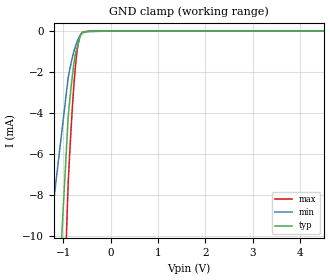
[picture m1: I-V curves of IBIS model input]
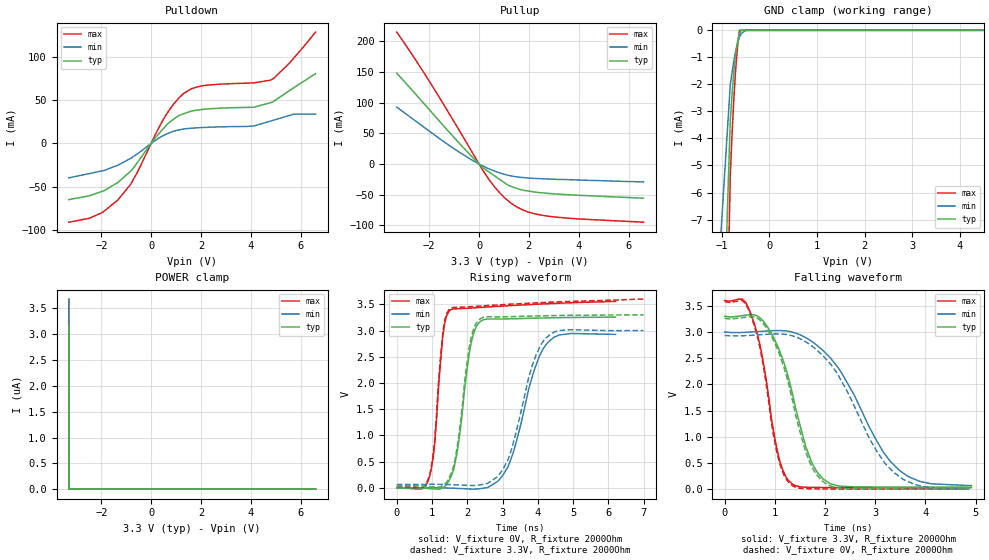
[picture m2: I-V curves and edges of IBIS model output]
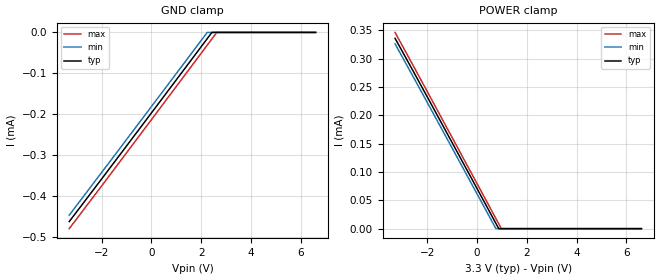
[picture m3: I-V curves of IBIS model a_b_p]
|Texas Instruments Incorporated
| Low-Voltage High-Speed Quadruple Differential Line Receiver
| With +/-15-kV IEC ESD
| Marketing part#   Digital Voltage Range   Package-type   #pins
| AM26LV32EIPWR   3.0V-3.6V   TSSOP   16
| AM26LV32EIPWRG4   3.0V-3.6V   TSSOP   16
| AM26LV32EIRGYR   3.0V-3.6V   VQFN   16
| AM26LV32EIRGYRG4   3.0V-3.6V   VQFN   16
| AM26LV32EID   3.0V-3.6V   SOIC   16
| AM26LV32EIDR   3.0V-3.6V   SOIC   16
[IBIS Ver]   4.1
[File name]   am26lv32e.ibs
[File Rev]   1.1
[Date]   11/01/2018
[Source]
| Texas Instruments Incorporated.
| Central Analog Engineering
| 12500 TI Blvd
| Dallas, TX -75243
[Notes]   Revision History:
| Rev 1.1: 11/01/2018
| - Add D package component
| Rev 1.0: 6/13/2013
| - Initial version of the model
| - Model generated from simulations in TISPICE
| - Model matched to SPICE simulation
| - C_comp although listed in numerical order of value are
|   obtained from varying PVT conditions. For PVT conditions for
|   each specific value refer the buffer description under
|   respective [Model]. IBIS model user is responsible for using
|   appropriate C_comp to simulate for Signal Integrity.
|*  EXCEPTION:   *
|*  - For model a_b_p and a_b_n ,There will be leakage in POWER Clamp   *
|*   IV table because of resistors R5,R14 connected to pad and GND Clamp   *
|*   IV table because of resistor R9 Connected to PAD.   *
|*  MODEL NOTE   *
|*  - This model is provided for use with both AM26LV32E and AM26LV32   *
|*   The silicon processes are different between these two parts, but only *
|*   one model is provided. The model is based on the AM26LV32E   *
|*   The accuracy of this model for AM26LV32 is limited and cannot be   *
|*   assured.
[Disclaimer]
| This model is designed as an aid for customers of Texas Instruments.
| TI and its licensors and suppliers make no warranties, either expressed
| or implied, with respect to this  model, including the warranties of
| merchantability or fitness for a particular purpose. The model is
| provided solely on an "as is" basis. The entire risk as to its quality
| and performance is with the customer.
[Copyright]
(C) Copyright 2018 Texas Instruments Incorporated.All rights reserved.
|   AM26LV32EPW
[Component]   AM26LV32EPW
[Manufacturer]   TI
[Package]   |16 TSSOP  -  PW  package
|   typ   min   max
R_pkg   0.19278   0.17677   0.20396
L_pkg   2.52752nH   2.29134nH   3.00408nH
C_pkg   0.42124pF   0.37067pF   0.48718pF
[Pin]  signal_name   model_name   R_pin   L_pin   C_pin
1   1B   a_b_n   0.17681   3.00040nH  0.48133pF
2   1A   a_b_p   0.19015   2.64657nH  0.48718pF
3   1Y   output   0.20396   2.39994nH  0.37179pF
4   G   input   0.19498   2.32104nH  0.37697pF
5   2Y   output   0.19142   2.29222nH  0.37501pF
6   2A   a_b_p   0.20200   2.38573nH  0.37069pF
7   2B   a_b_n   0.19014   2.64482nH  0.48580pF
8   GND   gnd   0.17006   2.94878nH  0.47879pF
9   3B   a_b_n   0.17677   3.00408nH  0.48145pF
10   3A   a_b_p   0.19010   2.64442nH  0.48578pF
11   3Y   output   0.20396   2.40233nH  0.37179pF
12   _G   input   0.19498   2.32182nH  0.37695pF
13   4Y   output   0.19142   2.29134nH  0.37502pF
14   4A   a_b_p   0.20200   2.38374nH  0.37067pF
15   4B   a_b_n   0.19019   2.64687nH  0.48695pF
16   VCC   power   0.18007   3.02750nH  0.48186pF
[Diff_pin]   inv_pin   vdiff   tdelay_typ   tdelay_min   tdelay_max
2   1   0.4   NA   NA   NA
6   7   0.4   NA   NA   NA
10   9   0.4   NA   NA   NA
14   15   0.4   NA   NA   NA
|   AM26LV32ERGY
[Component]   AM26LV32ERGY
[Manufacturer]   TI
[Package]   |16 VQFN   -  RGY package
|   typ   min   max
R_pkg   0.07133   0.06853   0.07388
L_pkg   1.07820nH   1.02485nH   1.12558nH
C_pkg   0.21525pF   0.20251pF   0.22285pF
[Pin]  signal_name   model_name   R_pin   L_pin   C_pin
1   1B   a_b_n   0.07388   1.12180nH  0.20251pF
2   1A   a_b_p   0.07293   1.10260nH  0.21277pF
3   1Y   output   0.07064   1.06987nH  0.22157pF
4   G   input   0.06991   1.04900nH  0.21124pF
5   2Y   output   0.06853   1.03338nH  0.20945pF
6   2A   a_b_p   0.07048   1.05873nH  0.22115pF
7   2B   a_b_n   0.07292   1.10180nH  0.22284pF
8   GND   gnd   0.07165   1.08613nH  0.22006pF
9   3B   a_b_n   0.07388   1.12558nH  0.21274pF
10   3A   a_b_p   0.07293   1.11070nH  0.21297pF
11   3Y   output   0.07064   1.06167nH  0.22136pF
12   _G   input   0.06991   1.05770nH  0.21146pF
13   4Y   output   0.06853   1.02485nH  0.20922pF
14   4A   a_b_p   0.07048   1.06724nH  0.22135pF
15   4B   a_b_n   0.07292   1.10994nH  0.22285pF
16   VCC   power   0.07593   1.15699nH  0.21430pF
[Diff_pin]   inv_pin   vdiff   tdelay_typ   tdelay_min   tdelay_max
2   1   0.4   NA   NA   NA
6   7   0.4   NA   NA   NA
10   9   0.4   NA   NA   NA
14   15   0.4   NA   NA   NA
|   AM26LV32EID
[Component]   AM26LV32EID
[Manufacturer]   TI
[Package]   |16 SOIC  -  D  package
|   typ   min   max
R_pkg   0.1097   0.0876   0.1214
L_pkg   2.6739n   1.8660n   3.6087n
C_pkg   0.5144p   0.3762p   0.7307p
[Pin]  signal_name   model_name   R_pin   L_pin   C_pin
1   1B   a_b_n   0.12139  3.60868n  0.72658p
2   1A   a_b_p   0.11814  2.95593n  0.55477p
3   1Y   output   0.11472  2.32743n  0.39842p
4   G   input   0.08877  1.89317n  0.37966p
5   2Y   output   0.08774  1.87902n  0.37623p
6   2A   a_b_p   0.11080  2.26165n  0.39561p
7   2B   a_b_n   0.11803  2.94830n  0.55794p
8   GND   gnd   0.11660  3.51494n  0.72633p
9   3B   a_b_n   0.12090  3.58634n  0.73071p
10   3A   a_b_p   0.11796  2.94490n  0.55767p
11   3Y   output   0.11472  2.32235n  0.39894p
12   _G   input   0.08886  1.88922n  0.37773p
13   4Y   output   0.08764  1.86597n  0.37772p
14   4A   a_b_p   0.11080  2.25473n  0.39472p
15   4B   a_b_n   0.11821  2.95453n  0.55408p
16   VCC   power   0.11952  3.57518n  0.72334p
[Diff_pin]   inv_pin   vdiff   tdelay_typ   tdelay_min   tdelay_max
2   1   0.4   NA   NA   NA
6   7   0.4   NA   NA   NA
10   9   0.4   NA   NA   NA
14   15   0.4   NA   NA   NA
| Models and submodels in the file (4): input (Input), output (3-state), a_b_p (Input), a_b_n (Input)
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|   input Model
[Model]   input
Model_type   Input
Vinl = 0.8
Vinh = 2.0
|   typ   min   max
|   (nom PVT)   (fast PVT)   (slow PVT)
C_comp   2.118e-12   2.106e-12   2.143e-12
| Where nom  PVT is Nominal Process, 3.3V, 27C
|   Fast PVT is Strong Process,  3.6V, -40C
|   Slow PVT is Weak Process,   3V, 125C
[Voltage Range]   3.3   3   3.6
|Junction Temperature
[Temperature Range]   27   125   -40
[Power Clamp Reference]   3.3   3   3.6
[GND Clamp Reference]   0   0   0
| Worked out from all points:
|   GND clamp passes 1 mA (typ) near -0.73 V on its own axis
[GND Clamp]
|   Voltage   I(typ)   I(min)   I(max)
-3.3V     -815.5mA   -63.93mA   -1.464A
-1.77V    -41.57mA   -19.44mA   -66.75mA
-897.6mV  -4.201mA   -2.276mA   -7.453mA
-853.2mV  -3.129mA   -1.753mA   -5.46mA
-810mV    -2.207mA   -1.299mA   -3.763mA
-774mV    -1.556mA   -971.7uA   -2.552mA
-738mV    -1.048mA   -694.3uA   -1.568mA
-702mV    -744.7uA   -469.8uA   -844.2uA
-669.6mV  -471.9uA   -316uA     -422.3uA
-633.6mV  -168.7uA   -195.4uA   -167.8uA
-586.8mV  -59.62uA   -89.39uA   -42.05uA
6.6V      0A         0A         0A
[POWER Clamp]
|   Voltage   I(typ)   I(min)   I(max)
-3.3V     0A         0A         0A
0V        0A         0A         0A
6.6V      0A         0A         0A
|   output Model
[Model]   output
Model_type   3-state
Polarity   Inverting
Vmeas = 1.65
Vref = 0
Cref = 15pF
Rref = 2000
|   typ   min   max
|   (nom PVT)   (fast PVT)   (slow PVT)
C_comp   3.751e-12   3.557e-12   4.057e-12
| Where nom  PVT is Nominal Process, 3.3V, 27C
|   Fast PVT is Strong Process,  3.6V, -40C
|   Slow PVT is Weak Process,   3V, 125C
[Voltage Range]   3.3   3   3.6
|Junction Temperature
[Temperature Range]   27   125   -40
[Pullup Reference]   3.3   3   3.6
[Pulldown Reference]   0   0   0
[Power Clamp Reference]   3.3   3   3.6
[GND Clamp Reference]   0   0   0
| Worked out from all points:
|   slope of the pulldown table from 0 to 0.495 V, typ, clamps not added: 28.7 ohm
|   slope of the pullup table from 0 to 0.495 V, typ, clamps not added: 31.5 ohm
|   GND clamp passes 1 mA (typ) near -0.72 V on its own axis
|   falling waveform, V_fixture 3.3V, R_fixture 2000Ohm: 20-80 % time 574ps typ, 1.02ns min, 377ps max; typ from 3.3 V to 0.038 V
|   rising waveform, V_fixture 0V, R_fixture 2000Ohm: 20-80 % time 363ps typ, 696ps min, 242ps max; typ from 0 V to 3.26 V
|   rising waveform, V_fixture 3.3V, R_fixture 2000Ohm: 20-80 % time 358ps typ, 671ps min, 246ps max; typ from 0.037 V to 3.3 V
|   falling waveform, V_fixture 0V, R_fixture 2000Ohm: 20-80 % time 563ps typ, 985ps min, 373ps max; typ from 3.26 V to 0 V
[Pulldown]
|   Voltage   I(typ)   I(min)   I(max)
-3.3V     -64.91mA   -39.78mA   -90.98mA
-2.486V   -60.54mA   -34.86mA   -86.52mA
-1.961V   -55.37mA   -31.68mA   -79.88mA
-1.345V   -45.31mA   -25.32mA   -65.66mA
-823.2mV  -32.07mA   -17.37mA   -47.39mA
584.4mV   20.16mA    10.34mA    32.12mA
1.312V    34.3mA     16.66mA    57.78mA
2.071V    39.2mA     18.38mA    66.61mA
4.125V    41.86mA    20.19mA    69.94mA
4.786V    47.01mA    25.76mA    73.04mA
5.742V    64.62mA    33.9mA     99.12mA
6.6V      80.6mA     33.9mA     128.6mA
[GND Clamp]
|   Voltage   I(typ)   I(min)   I(max)
-3.3V     -851.8mA   -106.7mA   -1.503A
-2.238V   -82.98mA   -41.6mA    -127.3mA
-825mV    -3.375mA   -2.041mA   -5.51mA
-801.6mV  -2.77mA    -1.749mA   -4.443mA
-776.4mV  -2.142mA   -1.436mA   -3.479mA
-749.1mV  -1.508mA   -1.138mA   -2.56mA
-726mV    -1.119mA   -890.4uA   -1.874mA
-675.6mV  -477.1uA   -503.2uA   -698.4uA
-628.8mV  -129.1uA   -249.4uA   0A
-597.3mV  -518.8nA   -135.5uA   0A
-498mV    -432.6nA   -2.253uA   0A
6.6V      0A         0A         0A
[Pullup]
|   Voltage   I(typ)   I(min)   I(max)
-3.3V     148mA      92.72mA    215mA
-2.17V    96.59mA    58.75mA    146.2mA
-825mV    35.29mA    20.19mA    57mA
19.8mV    -787.1uA   -413uA     -1.283mA
400.8mV   -13.03mA   -7.878mA   -25.36mA
850.8mV   -25.77mA   -14.78mA   -47.91mA
1.29V     -36.59mA   -19.41mA   -63.98mA
1.52V     -39.95mA   -20.98mA   -70.12mA
1.995V    -44.22mA   -22.92mA   -78.54mA
2.622V    -47.36mA   -24.22mA   -84.21mA
4.123V    -51.27mA   -26.26mA   -89.85mA
6.6V      -55.74mA   -29.32mA   -94.86mA
[POWER Clamp]
|   Voltage   I(typ)   I(min)   I(max)
-3.3V     3.161uA    3.682uA    3.68uA
-3.297V   1.724uA    545.5nA    2.147uA
-3.293V   0A         218.2nA    306.6nA
-3.293V   0A         163.7nA    0A
-3.291V   0A         0A         0A
6.6V      0A         0A         0A
[Ramp]
R_load = 2000
|   typ   min   max
dV/dt_r   1.95542/3.608e-10   1.75784/6.87955e-10   2.14457/2.43246e-10
dV/dt_f   1.95755/5.69827e-10   1.76035/1.01256e-09   2.14363/3.74807e-10
[Falling Waveform]
V_fixture = 3.3V
V_fixture_min = 3V
V_fixture_max = 3.6V
R_fixture = 2000Ohm
|   Time   V(typ)   V(min)   V(max)
0s        3.3V       3V         3.6V
348ps     3.311V     2.991V     3.628V
512ps     3.33V      2.999V     3.374V
732ps     3.245V     3.012V     2.614V
1.096ns   2.633V     3.026V     544.4mV
1.36ns    1.78V      2.994V     92.08mV
1.722ns   540.9mV    2.829V     34.87mV
2.1ns     107.5mV    2.513V     30.77mV
3.48ns    39.83mV    360.4mV    27.35mV
4.918ns   37.7mV     70.1mV     27.48mV
[Rising Waveform]
V_fixture = 0V
V_fixture_min = 0V
V_fixture_max = 0V
R_fixture = 2000Ohm
|   Time   V(typ)   V(min)   V(max)
0s        316.8pV    601.3pV    223.4pV
932ps     -13.59mV   4.127mV    218.1mV
1.298ns   2.197mV    1.585mV    2.857V
1.488ns   147.2mV    -2.535mV   3.374V
1.742ns   817.9mV    -9.586mV   3.417V
2.106ns   2.76V      -22.17mV   3.428V
2.358ns   3.169V     -14.47mV   3.439V
3.154ns   3.222V     403.4mV    3.472V
4.258ns   3.241V     2.756V     3.51V
6.198ns   3.256V     2.927V     3.555V
[Rising Waveform]
V_fixture = 3.3V
V_fixture_min = 3V
V_fixture_max = 3.6V
R_fixture = 2000Ohm
|   Time   V(typ)   V(min)   V(max)
0s        37.23mV    65.79mV    27.12mV
932ps     23.97mV    69.69mV    252.1mV
1.054ns   18.09mV    69.82mV    764.8mV
1.306ns   46.9mV     66.84mV    2.963V
1.536ns   271.9mV    61.87mV    3.429V
2.094ns   2.819V     46.9mV     3.455V
2.35ns    3.216V     57.12mV    3.466V
3.12ns    3.263V     492.9mV    3.498V
4.21ns    3.282V     2.85V      3.535V
6.992ns   3.3V       3V         3.6V
[Falling Waveform]
V_fixture = 0V
V_fixture_min = 0V
V_fixture_max = 0V
R_fixture = 2000Ohm
|   Time   V(typ)   V(min)   V(max)
0s        3.261V     2.934V     3.575V
346ps     3.273V     2.927V     3.604V
506ps     3.291V     2.935V     3.359V
718ps     3.216V     2.949V     2.627V
1.088ns   2.581V     2.961V     515.9mV
1.356ns   1.678V     2.925V     63.63mV
1.698ns   508.1mV    2.762V     8.037mV
2.086ns   68.9mV     2.413V     3.675mV
3.36ns    3mV        327.6mV    198.8uV
4.872ns   465.8uV    3.439mV    350.3uV
|   a_b Model
[Model]   a_b_p
Model_type   Input
Vinl = 0.8
Vinh = 2.0
|   typ   min   max
|   (nom PVT)   (fast PVT)   (slow PVT)
C_comp   3.305e-12   3.305e-12   3.478e-12
| Where nom  PVT is Nominal Process, 3.3V, 27C
|   Fast PVT is Strong Process,  3.6V, -40C
|   Slow PVT is Weak Process,   3V, 125C
[Voltage Range]   3.3   3   3.6
|Junction Temperature
[Temperature Range]   27   125   -40
[Power Clamp Reference]   3.3   3   3.6
[GND Clamp Reference]   0   0   0
[GND Clamp]
|   Voltage   I(typ)   I(min)   I(max)
-3.3V     -462.8uA   -447.2uA   -480.1uA
2.244V    -15.34uA   -171.3nA   -31.25uA
2.432V    -79.03nA   0A         -15.94uA
2.632V    0A         0A         0A
6.6V      0A         0A         0A
[POWER Clamp]
|   Voltage   I(typ)   I(min)   I(max)
-3.3V     335.9uA    326.3uA    346.4uA
753mV     9.241uA    71.41nA    17.82uA
864.6mV   188.7nA    0A         8.743uA
972mV     0A         0A         0A
6.6V      0A         0A         0A
